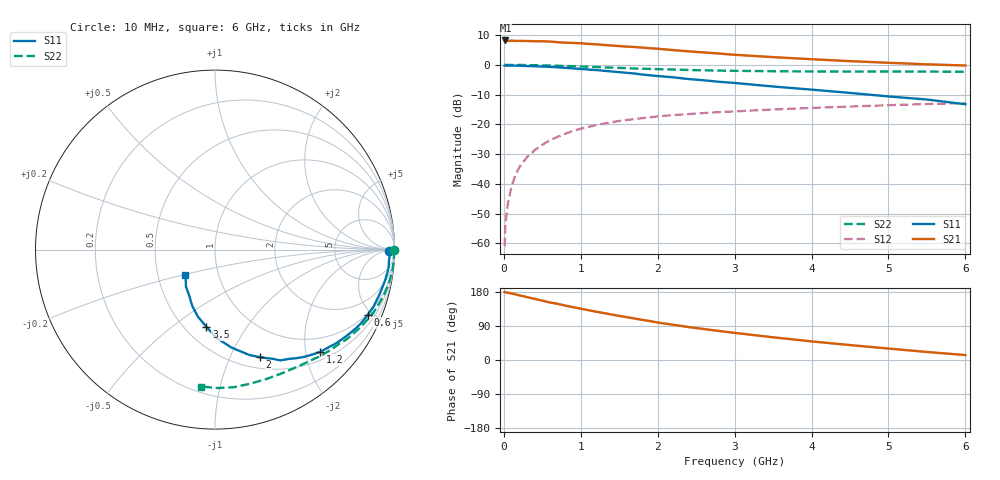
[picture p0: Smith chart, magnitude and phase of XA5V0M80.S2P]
! SIEMENS Discrete & RF Semiconductors
! BFY180
! Si NPN RF Bipolar Junction Transistor in MICRO-X
! VCE = 5 V  IC = 0.8 mA
! Common Emitter S-Parameters:  May  1997
# GHz  S  MA  R  50
!  f  S11  S21  S12  S22
! GHz  MAG  ANG  MAG  ANG  MAG  ANG  MAG  ANG
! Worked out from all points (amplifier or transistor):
!   36 points, 10 MHz to 6 GHz, reference 50 ohm
!   highest |S21| = 8.2 dB at 20 MHz (marker M1)
!   |S21| within 3 dB of that: start of sweep to 2.095 GHz
!   unconditionally stable (mu >= 1): 4.488 GHz to end of sweep
!   at 250 MHz: K = 0.05, MSG = 20.3 dB, |S12| = -32.7 dB
!   at 1.4 GHz: K = 0.45, MSG = 12.9 dB, |S12| = -19.3 dB
!   at 6 GHz: K = 1.04, MAG = 5.1 dB, |S12| = -12.8 dB
!   S11 on the Smith chart (normalised r, x): 10 MHz: 68, -12; 600 MHz: 0.92, -4.70; 1.2 GHz: 0.67, -2.30; 2 GHz: 0.63, -1.30; 3.5 GHz: 0.63, -0.67; 6 GHz: 0.69, -0.21
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0.01  0.9719 -0.3  2.553 179.4  0.0009 86.6  0.9981 -0.2
0.02  0.9729 -1.1  2.573 178.7  0.0021 95.3  0.9999 -0.6
0.05  0.9743 -1.5  2.523 177.7  0.0045 87.7  0.9975 -1.2
0.1  0.9711 -3.9  2.553 175.5  0.009 89.2  0.9983 -2.5
0.15  0.9728 -5.9  2.527 173.3  0.0142 86.8  0.9979 -3.8
0.2  0.9683 -7.9  2.534 170.7  0.0189 83.5  0.9964 -5.0
0.4  0.9488 -15.6  2.497 161.4  0.0369 79.0  0.989 -9.8
0.5  0.9389 -19.7  2.499 156.6  0.0455 76.0  0.9825 -12.3
0.6  0.9258 -23.2  2.461 151.7  0.0542 73.2  0.9757 -14.6
0.9  0.8735 -33.8  2.34 139.5  0.0778 65.3  0.9504 -21.5
1.1  0.8353 -40.6  2.254 131.4  0.0909 60.3  0.9295 -25.7
1.2  0.8181 -44.1  2.216 127.5  0.0972 57.9  0.9205 -27.9
1.7  0.7165 -59.5  1.997 109.5  0.1228 48.5  0.8694 -36.9
2  0.6492 -67.3  1.868 98.9  0.1363 43.6  0.8483 -41.9
2.2  0.6188 -71.8  1.772 93.0  0.1435 40.6  0.836 -45.1
2.4  0.578 -76.8  1.688 87.0  0.1489 37.9  0.8206 -48.0
2.8  0.5197 -84.7  1.55 76.5  0.1607 33.5  0.8018 -53.3
3.5  0.4334 -96.4  1.35 59.9  0.1781 26.7  0.7824 -62.4
4  0.3841 -104.5  1.245 49.1  0.1892 22.3  0.7755 -68.8
4.5  0.3382 -112.0  1.156 39.4  0.1994 18.2  0.7723 -75.4
5.5  0.2617 -128.2  1.022 21.2  0.2199 10.1  0.7714 -89.0
6  0.2182 -138.9  0.977 13.0  0.2279 5.9  0.7668 -95.9
